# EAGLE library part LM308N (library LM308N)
Operational Amplifiers - Op Amps Source: Datasheet
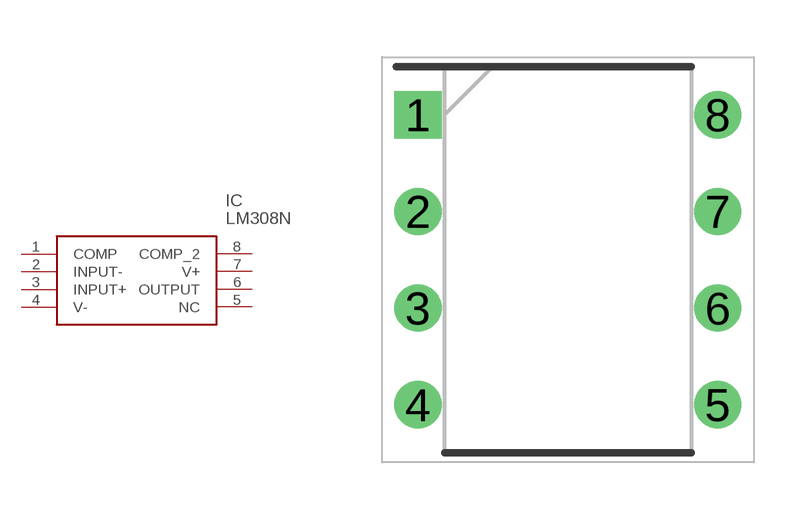
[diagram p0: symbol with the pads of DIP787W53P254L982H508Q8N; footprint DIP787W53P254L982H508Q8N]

Designator prefix IC

## LM308N (Description: Operational Amplifiers - Op Amps; Height: 5.08mm; Manufacturer_Name: Texas Instruments; Manufacturer_Part_Number: LM308N; Mouser_Part_Number: N/A; Mouser_Price-Stock: https://www.mouser.com/Search/Refine.aspx?Keyword=N%2FA)  [DIP787W53P254L982H508Q8N]
1  COMP
2  INPUT-
3  INPUT+
4  V-
5  NC  nc
6  OUTPUT
7  V+
8  COMP_2

## Footprint DIP787W53P254L982H508Q8N (pad centres in mm)
N08E-1
drill 0.733 pad 1.133 square: 1 -3.937,3.81
drill 0.733 pad 1.133: 2 -3.937,1.27; 3 -3.937,-1.27; 4 -3.937,-3.81; 5 3.937,-3.81; 6 3.937,-1.27; 7 3.937,1.27; 8 3.937,3.81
